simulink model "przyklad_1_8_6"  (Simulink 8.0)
settings: Solver=ode45  StartTime=0.0  StopTime=0.1  RelTol=1e-11
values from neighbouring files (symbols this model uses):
  C1 = 4.7*1.E-3    (= 0.0047)    [przykl_2_8_par.m]
  C2 = 22.0*1.E-6    (= 2.2e-05)    [przykl_2_8_par.m]
  L = 2.5    [przykl_2_8_par.m]
  R1 = 10.0    (= 10)    [przykl_2_8_par.m]
  R2 = 500.0    (= 500)    [przykl_2_8_par.m]

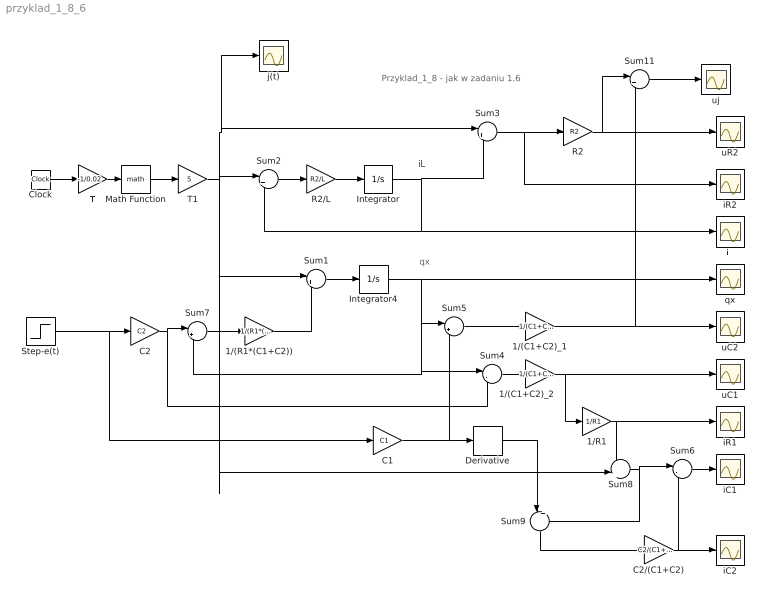
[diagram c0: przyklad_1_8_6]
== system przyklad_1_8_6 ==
  note: qx
  note: iL
  note: Przyklad_1_8 - jak w zadaniu 1.6
  1/(C1+C2)_1 : Gain  Gain=1/(C1+C2)
  1/(C1+C2)_2 : Gain  Gain=1/(C1+C2)
  1/(R1*(C1+C2)) : Gain  Gain=1/(R1*(C1+C2))
  1/R1 : Gain  Gain=1/R1
  C1 : Gain  Gain=C1
  C2 : Gain  Gain=C2
  C2/(C1+C2) : Gain  Gain=C2/(C1+C2)
  Clock : Clock
  Derivative : Derivative
  Integrator : Integrator
  Integrator4 : Integrator
  Math Function : Math
  R2 : Gain  Gain=R2
  R2/L : Gain  Gain=R2/L
  Step-e(t) : Step  Time=0  After=48  SampleTime=0
  Sum{1,5,9,11} (4 alike) : Sum  Inputs=|++
  Sum2 : Sum  Inputs=|+-
  Sum3 : Sum  Inputs=|+-
  Sum4 : Sum  Inputs=|-+
  Sum6 : Sum  Inputs=|-+
  Sum7 : Sum  Inputs=|+-
  Sum8 : Sum  Inputs=+|+
  T : Gain  Gain=-1/0.02
  T1 : Gain  Gain=5
  iC1 : Scope
  iC2 : Scope
  iL : Scope
  iR1 : Scope
  iR2 : Scope
  j(t) : Scope
  qx : Scope
  uC1 : Scope
  uC2 : Scope
  uR2 : Scope
  uj : Scope
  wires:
  Sum2/1 -> R2/L/1
  Sum1/1 -> Integrator4/1
  Integrator4/1 -> Sum7/2, Sum4/1, Sum5/1, qx/1
  Integrator/1 -> iL/1, Sum2/2, Sum3/2
  1/(R1*(C1+C2))/1 -> Sum1/2
  Clock/1 -> T/1
  Sum3/1 -> iR2/1, R2/1
  Sum4/1 -> 1/(C1+C2)_2/1
  Sum5/1 -> 1/(C1+C2)_1/1
  1/(C1+C2)_1/1 -> Sum11/2, uC2/1
  1/(C1+C2)_2/1 -> 1/R1/1, uC1/1
  1/R1/1 -> Sum8/1, iR1/1
  C2/1 -> Sum4/2, Sum7/1
  C1/1 -> Sum5/2, Derivative/1
  Derivative/1 -> Sum9/1
  C2/(C1+C2)/1 -> iC2/1, Sum6/2
  R2/L/1 -> Integrator/1
  R2/1 -> Sum11/1, uR2/1
  Sum7/1 -> 1/(R1*(C1+C2))/1
  Sum8/1 -> Sum9/2, Sum6/1
  Sum9/1 -> C2/(C1+C2)/1
  Sum6/1 -> iC1/1
  Step-e(t)/1 -> C1/1, C2/1
  Sum11/1 -> uj/1
  Math Function/1 -> T1/1
  T/1 -> Math Function/1
  T1/1 -> Sum8/2, Sum1/1, Sum2/1, j(t)/1, Sum3/1
